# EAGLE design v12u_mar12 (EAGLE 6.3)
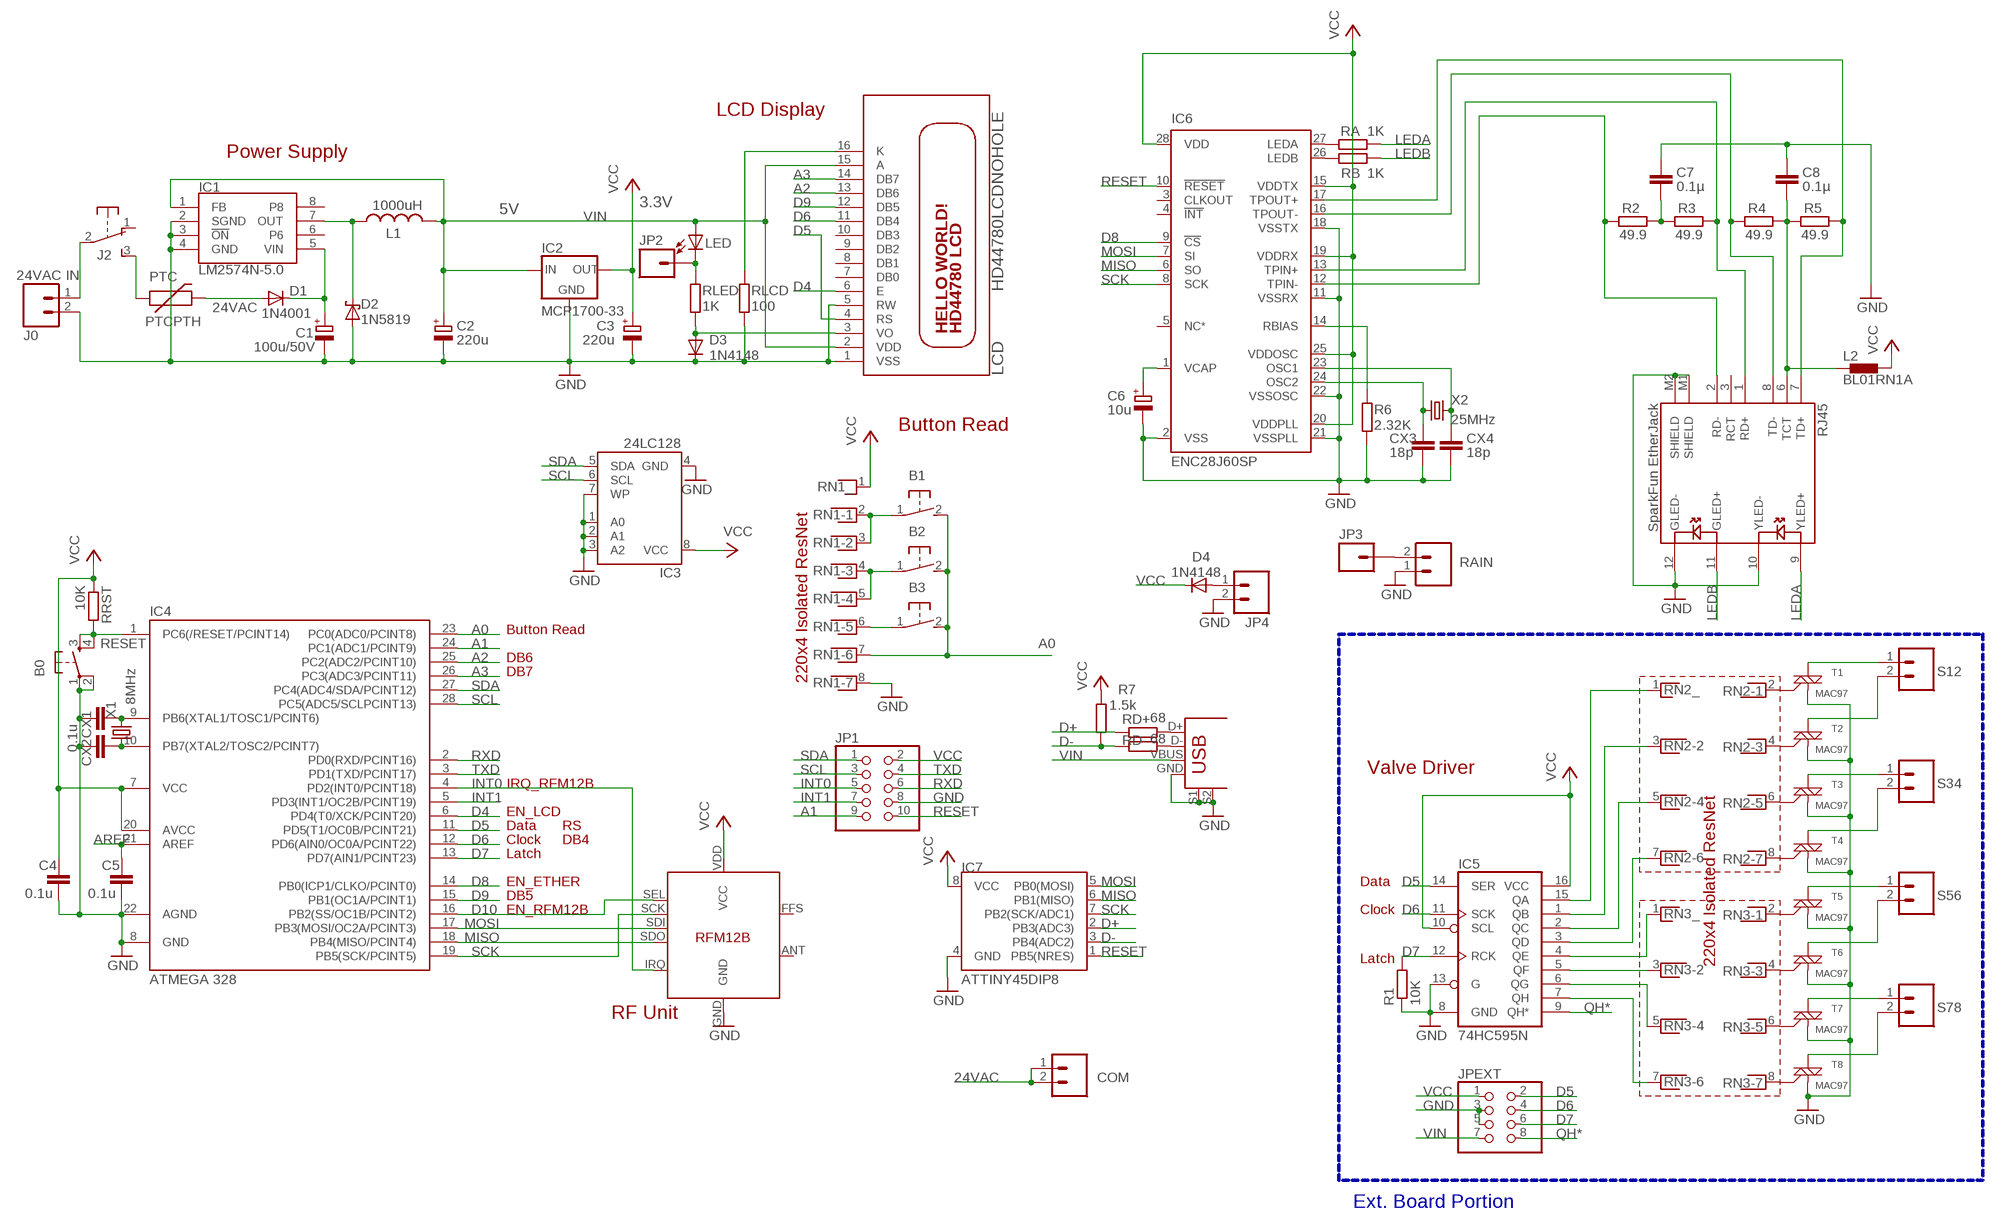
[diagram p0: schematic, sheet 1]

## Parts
B0  TAC_SWITCHPTH  [TACTILE-PTH]
B1  31-XX  [B3F-31XX]
B2  31-XX  [B3F-31XX]
B3  31-XX  [B3F-31XX]
C1  100u/50V  CPOL-EUE3.5-8  [E3,5-8]
C2  220u  CPOL-EUE2-5  [E2-5]
C3  220u  CPOL-EUE2-5  [E2-5]
C4  0.1u  C-EU025-024X044  [C025-024X044]
C5  0.1u  C-EU025-024X044  [C025-024X044]
C6  10u  CPOL-EUE1.8-4  [E1,8-4]
C7  0.1µ  C-EU025-024X044  [C025-024X044]
C8  0.1µ  C-EU025-024X044  [C025-024X044]
COM  M025MM  [SCREWTERMINAL-5MM-2]
CX1  0.1u  C-EU025-024X044  [C025-024X044]
CX2  0.1u  C-EU025-024X044  [C025-024X044]
CX3  18p  C-EU025-024X044  [C025-024X044]
CX4  18p  C-EU025-024X044  [C025-024X044]
D1  1N4001  DIODE-DO41-7.6  [DO41-7.6]
D2  1N5819  1N5817-B  [DO41-7.6]
D3  1N4148  1N4148DO35-7  [DO35-7]
D4  1N4148  1N4148DO35-7  [DO35-7]
IC1  LM2574N-5.0  LM2574N  [DIL08]
IC2  MCP1700-33  MCP1700INLINE  [TO92-INLINE]
IC3  24LC128  AT24CP  [DIL08]
IC4  ATMEGA 328  ATMEGA48/88/168-PU  [DIL28-3]
IC5  74HC595N  74LS595N  [DIL16]
IC6  ENC28J60SP  [DIL28-3]
IC7  ATTINY45DIP8  [DIP08]
IC8  RFM12B  [RFM12B]
J0  24VAC IN  M025MM  [SCREWTERMINAL-5MM-2]
J2  EG1206  [EG1206]
JP1  PINHD-2X5  [2X05]
JP2  M01PTH  [1X01]
JP3  M01PTH  [1X01]
JP4  M02PTH  [1X02]
JPEXT  PINHD-2X4  [2X04]
L1  1000uH  L-US6000-XXX-RC  [6000-XXXX-RC]
L2  BL01RN1A  [BL01RN1A]
LCD  HD44780LCDNOHOLE  [LCD1602A]
LED  POWERLED  LED3MM  [LED3MM]
PTC  PTCPTH  [PTC]
R1  10K  R-EU_0204/7  [0204/7]
R2  49.9  R-EU_0204/7  [0204/7]
R3  49.9  R-EU_0204/7  [0204/7]
R4  49.9  R-EU_0204/7  [0204/7]
R5  49.9  R-EU_0204/7  [0204/7]
R6  2.32K  R-EU_0204/7  [0204/7]
R7  1.5k  R-EU_0204/7  [0204/7]
RA  1K  R-EU_0204/7  [0204/7]
RAIN  M025MM  [SCREWTERMINAL-5MM-2]
RB  1K  R-EU_0204/7  [0204/7]
RD+  68  R-EU_0204/7  [0204/7]
RD-  68  R-EU_0204/7  [0204/7]
RJ45  SparkFun EtherJack  MAGJACK  [MAGJACK]
RLCD  100  R-EU_0204/7  [0204/7]
RLED  1K  R-EU_0204/7  [0204/7]
RN1  RNX7  [RN-8]
RN2  RNX7  [RN-8]
RN3  RNX7  [RN-8]
RRST  10K  R-EU_0204/7  [0204/7]
S12  M025MM  [SCREWTERMINAL-5MM-2]
S34  M025MM  [SCREWTERMINAL-5MM-2]
S56  M025MM  [SCREWTERMINAL-5MM-2]
S78  M025MM  [SCREWTERMINAL-5MM-2]
T1  MAC97  LX807DE  [TO-92]
T2  MAC97  LX807DE  [TO-92]
T3  MAC97  LX807DE  [TO-92]
T4  MAC97  LX807DE  [TO-92]
T5  MAC97  LX807DE  [TO-92]
T6  MAC97  LX807DE  [TO-92]
T7  MAC97  LX807DE  [TO-92]
T8  MAC97  LX807DE  [TO-92]
USB  USB+SHIELD  [USB-B-PTH]
X1  8MHz  CRYSTALTC26V  [TC26V]
X2  25MHz  CRYSTALHC49US  [HC49US]

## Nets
24VAC [power]: COM.1 COM.2 D1.A PTC.P$2
A0: B1.2(S) B2.2(S) B3.2(S) IC4.23(PC0(ADC0/PCINT8)) RN1.7
A1: IC4.24(PC1(ADC1/PCINT9)) JP1.9
A2: IC4.25(PC2(ADC2/PCINT10)) LCD.13(DB6)
A3: IC4.26(PC3(ADC3/PCINT11)) LCD.14(DB7)
AREF: C5.1 IC4.21(AREF)
D4: IC4.6(PD4(T0/XCK/PCINT20)) LCD.6(E)
D5: IC4.11(PD5(T1/OC0B/PCINT21)) IC5.14(SER) JPEXT.2 LCD.4(RS)
D6: IC4.12(PD6(AIN0/OC0A/PCINT22)) IC5.11(SCK) JPEXT.4 LCD.11(DB4)
D7: IC4.13(PD7(AIN1/PCINT23)) IC5.12(RCK) JPEXT.6 R1.2
D8: IC4.14(PB0(ICP1/CLKO/PCINT0)) IC6.9(!CS)
D9: IC4.15(PB1(OC1A/PCINT1)) LCD.12(DB5)
D10: IC4.16(PB2(SS/OC1B/PCINT2)) IC8.SEL
D+: IC7.2(PB3(ADC3)) RD+.1
D-: IC7.3(PB4(ADC2)) R7.1 RD-.1
GND [power]: B0.1 B0.2 C1.- C2.- C3.- C4.2 C5.2 C6.- C7.1 C8.1 CX1.1 CX2.1 CX3.2 CX4.2 D2.A D3.C IC1.2(SGND) IC1.3(!ON) IC1.4(GND) IC2.1(GND) IC3.1(A0) IC3.2(A1) IC3.3(A2) IC3.4(GND) IC3.7(WP) IC4.8(GND) IC4.22(AGND) IC5.8(GND) IC5.13(G) IC6.2(VSS) IC6.11(VSSRX) IC6.18(VSSTX) IC6.21(VSSPLL) IC6.22(VSSOSC) IC7.4(GND) IC8.GND J0.2 JP1.8 JP4.2 JPEXT.3 JPEXT.5 LCD.1(VSS) LCD.5(RW) R1.1 R6.2 RAIN.1 RJ45.10(YLED-) RJ45.12(GLED-) RJ45.M1(SHIELD) RJ45.M2(SHIELD) RLCD.2 RN1.8 T1.1(M1) T2.1(M1) T3.1(M1) T4.1(M1) T5.1(M1) T6.1(M1) T7.1(M1) T8.1(M1) USB.GND USB.S1 USB.S2
INT0: IC4.4(PD2(INT0/PCINT18)) IC8.IRQ JP1.5
INT1: IC4.5(PD3(INT1/OC2B/PCINT19)) JP1.7
LEDA: RA.2 RJ45.9(YLED+)
LEDB: RB.2 RJ45.11(GLED+)
MISO: IC4.18(PB4(MISO/PCINT4)) IC6.6(SO) IC7.6(PB1(MISO)) IC8.SDO
MOSI: IC4.17(PB3(MOSI/OC2A/PCINT3)) IC6.7(SI) IC7.5(PB0(MOSI)) IC8.SDI
N$2: CX1.2 IC4.9(PB6(XTAL1/TOSC1/PCINT6)) X1.2
N$3: RN2.2 T1.2(G)
N$4: IC5.5(QF) RN3.3
N$5: IC5.6(QG) RN3.5
N$6: J0.1 J2.2(P)
N$7: IC5.7(QH) RN3.7
N$8: CX2.2 IC4.10(PB7(XTAL2/TOSC2/PCINT7)) X1.1
N$9: C1.+ D1.C IC1.5(VIN)
N$10: IC5.4(QE) RN3.1
N$11: IC5.3(QD) RN2.7
N$12: IC5.2(QC) RN2.5
N$13: IC5.1(QB) RN2.3
N$14: IC5.15(QA) RN2.1
N$15: RN2.4 T2.2(G)
N$16 [power]: S12.1 T1.3(M2)
N$17 [power]: S12.2 T2.3(M2)
N$18 [power]: S34.1 T3.3(M2)
N$19: RN2.6 T3.2(G)
N$20 [power]: S34.2 T4.3(M2)
N$21: RN2.8 T4.2(G)
N$22 [power]: S56.1 T5.3(M2)
N$23 [power]: S56.2 T6.3(M2)
N$24 [power]: S78.1 T7.3(M2)
N$25 [power]: S78.2 T8.3(M2)
N$26: RN3.2 T5.2(G)
N$27: RN3.4 T6.2(G)
N$28: RN3.6 T7.2(G)
N$29: RN3.8 T8.2(G)
N$30: C8.2 L2.1 R4.2 R5.1 RJ45.6(TCT)
N$31: J2.3(S) PTC.P$1
N$32: B1.1(P) RN1.2 RN1.3
N$33: B3.1(P) RN1.6
N$34: IC6.27(LEDA) RA.1
N$35: B2.1(P) RN1.4 RN1.5
N$36: IC6.26(LEDB) RB.1
N$37: JP2.1 LED.K(C) RLED.1
N$38: RD+.2 USB.D+
N$39: D3.A LCD.3(VO) RLED.2
N$40 [power]: D2.C IC1.7(OUT) L1.1
N$41: IC6.17(TPOUT+) R5.2 RJ45.7(TD+)
N$42: IC6.16(TPOUT-) R4.1 RJ45.8(TD-)
N$43: IC6.13(TPIN+) R3.2 RJ45.1(RD+)
N$44: IC6.12(TPIN-) R2.1 RJ45.2(RD-)
N$45: RD-.2 USB.D-
N$46: D4.A JP4.1
N$47: JP3.1 RAIN.2
N$48: LCD.16(K) RLCD.1
N$50: C6.+ IC6.1(VCAP)
N$51: IC6.14(RBIAS) R6.1
N$52: CX3.1 IC6.24(OSC2) X2.1
N$53: CX4.1 IC6.23(OSC1) X2.2
N$54: C7.2 R2.2 R3.1
QH*: IC5.9(QH*) JPEXT.8
RESET: B0.3 B0.4 IC4.1(PC6(/RESET/PCINT14)) IC6.10(!RESET) IC7.1(PB5(NRES)) JP1.10 RRST.2
RXD: IC4.2(PD0(RXD/PCINT16)) JP1.6
SCK: IC4.19(PB5(SCK/PCINT5)) IC6.8(SCK) IC7.7(PB2(SCK/ADC1)) IC8.SCK
SCL: IC3.6(SCL) IC4.28(PC5(ADC5/SCLPCINT13)) JP1.3
SDA: IC3.5(SDA) IC4.27(PC4(ADC4/SDA/PCINT12)) JP1.1
TXD: IC4.3(PD1(TXD/PCINT17)) JP1.4
VCC: C3.+ C4.1 D4.C IC2.3(OUT) IC3.8(VCC) IC4.7(VCC) IC4.20(AVCC) IC5.10(SCL) IC5.16(VCC) IC6.15(VDDTX) IC6.19(VDDRX) IC6.20(VDDPLL) IC6.25(VDDOSC) IC6.28(VDD) IC7.8(VCC) IC8.VDD(VCC) JP1.2 JPEXT.1 L2.2 R7.2 RN1.1 RRST.1
VIN: C2.+ IC1.1(FB) IC2.2(IN) JPEXT.7 L1.2 LCD.2(VDD) LCD.15(A) LED.A USB.VBUS
Unconnected: IC1.6 IC1.8 IC6.3(CLKOUT) IC6.4(!INT) IC6.5(NC*) IC8.ANT IC8.FFS J2.1(O) LCD.7(DB0) LCD.8(DB1) LCD.9(DB2) LCD.10(DB3) RJ45.3(RCT)

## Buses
B$1

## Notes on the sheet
- LCD Display
- Power Supply
- 3.3V
- 5V
- Button Read
- Button Read
- DB6
- DB7
- 220x4 Isolated ResNet
- Valve Driver
- IRQ_RFM12B
- 220x4 Isolated ResNet
- EN_LCD
- Data | RS
- Clock | DB4
- Latch
- EN_ETHER | Data
- DB5
- EN_RFM12B | Clock
- Latch
- RF Unit
- Ext. Board Portion

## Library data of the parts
B0 = SparkFun:TAC_SWITCH: Momentary Switch Button commonly used for reset or general input. Spark Fun Electronics SKU : COM-00097
B1-B3 = adafruit:31-XX: OMRON SWITCH
C1-C3 C6 = resistor:CPOL-EU: POLARIZED CAPACITOR, European symbol
C4 C5 CX1 CX2 = rcl:C-EU: CAPACITOR, European symbol
C7 C8 CX3 CX4 = resistor:C-EU: CAPACITOR, European symbol
COM J0 JP4 RAIN S12 S34 S56 S78 = SparkFun:M02: Header 2
D1 = diode:DIODE-: DIODE
D2 = diode:1N581*: 1.0A SCHOTTKY BARRIER RECTIFIER
D3 D4 = diode:1N4148: DIODE
IC1 = linear-technology:LM2574N
IC2 = adafruit:MCP1700: VOLTAGE REGULATOR
IC3 = atmel:AT24C*: 2-wire serial EEPROM; MPN: AT24C1024BW-SH-B; OC_FARNELL: 1362646; OC_NEWARK: 03P2044
IC4 = atmega8:ATMEGA48/88/168-PU
IC5 = SparkFun:74*595: 8-bit SHIFT REGISTER, output latch
IC6 = microchip:ENC28J60: Stand-Alone Ethernet Controller with SPI Interface Source: http://ww1.microchip.com/downloads/en/DeviceDoc/39662c.pdf; MF: MICROCHIP; MPN: ENC28J60/SP; OC_FARNELL: 1084619; OC_NEWARK: 96K3661
IC7 = SparkFun:ATTINY45: Atmel ATTiny45
IC8 = JeeLabs:RFM12B
J2 = adafruit:EG1206
JP1 = pinhead:PINHD-2X5: PIN HEADER
JP2 JP3 = SparkFun:M01: Header 1
JPEXT = pinhead:PINHD-2X4: PIN HEADER
L1 = rcl:L-US: INDUCTOR, American symbol
L2 = inductors:BL0: Noise Suppression Products/EMI Suppression Filters, Lead EMIFIL(R) Inductor Type
LCD = adafruit:HD44780LCD: HD44780 LCD Standard character type LCDs, available in sizes from 8x1 to 40x4!
LED = adafruit:LED: LED
PTC = SparkFunNew:PTC: Resettable Fuse PTC
R1-R7 RA RB RD+ RD- RLCD RLED RRST = rcl:R-EU_: RESISTOR, European symbol
RJ45 = SparkFunNew:MAGJACK
RN1-RN3 = resistor-net:RNX7: RESISTOR NETWORK; OC_FARNELL: unknown; OC_NEWARK: unknown
T1-T8 = SparkFun:LX807DE: LX807DE Triac http://www.littelfuse.com/data/en/Data_Sheets/Littelfuse_Triac_LX8.pdf
USB = SparkFunNew:USB+SHIELD: USB+Shield USB connector with shield pins connectable
X1 = crystal:CRYSTAL: CRYSTAL; OC_FARNELL: unknown; OC_NEWARK: unknown
X2 = SparkFun:CRYSTAL: Crystals

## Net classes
0 default: width 0.406 mm, clearance 0.203 mm
1 power: width 0.813 mm, clearance 0.203 mm

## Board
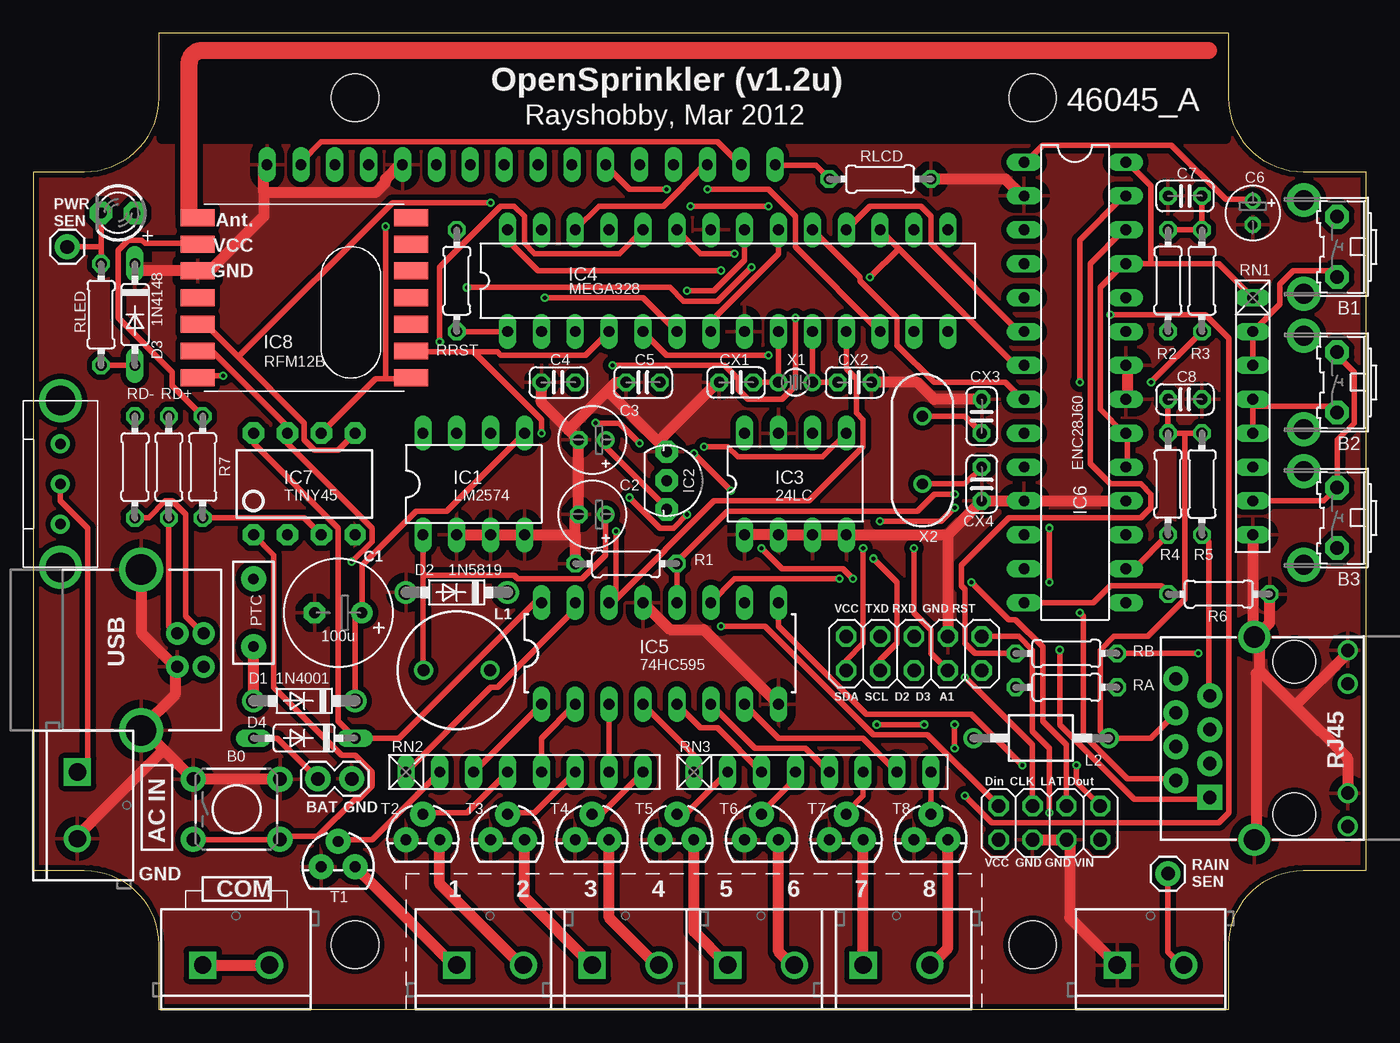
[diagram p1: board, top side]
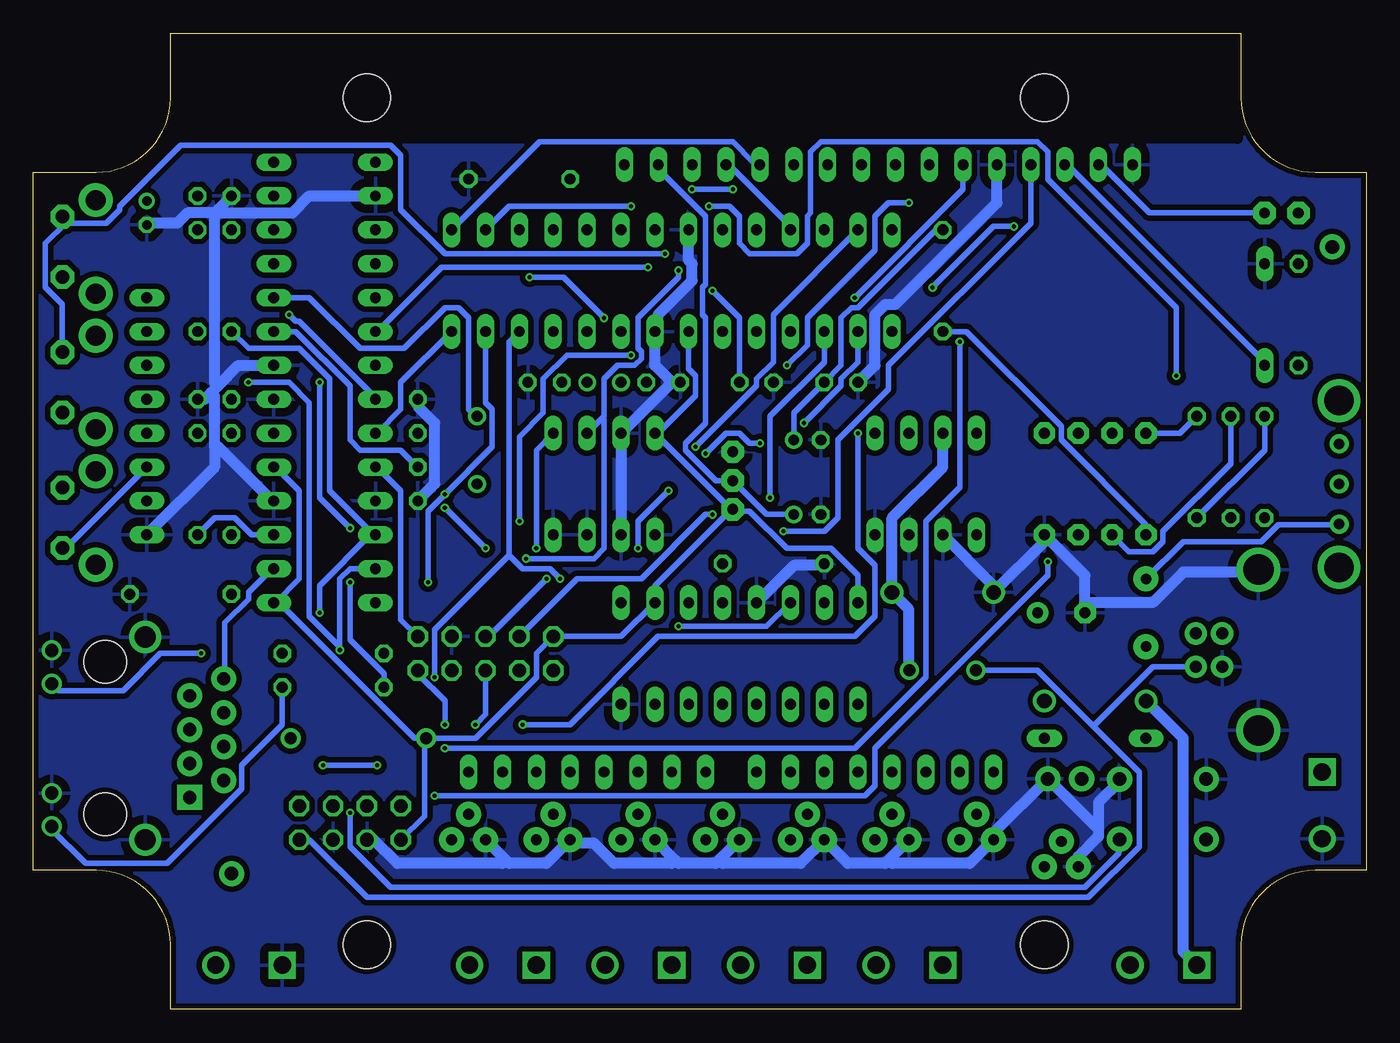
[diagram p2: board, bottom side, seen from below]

Size 99.95 x 73.15 mm. Coordinates in mm from the lower left corner, seen from the top.
Outline: 9.4,0 89.66,0 89.66,4.83 arc-90 95.25,10.41 99.95,10.41 99.95,62.74 95.25,62.74 arc-90 89.66,68.33 89.66,73.15 9.4,73.15 9.4,68.33 arc-90 3.81,62.74 0,62.74 0,10.41 3.81,10.41 arc-90 9.4,4.83 9.4,0
Copper layers (1*16): Top 0.035mm / dielectric 1.5mm / Bottom 0.035mm
Design rules "Fusion_eagle_rule_v1.1 *": minimum track width 6mil, minimum drill 12mil, track to track 6mil, track to pad 6mil, pad to pad 8mil, via to via 8mil, smd to smd 0mil, copper to edge 10mil, drill to drill 10mil, minimum pad ring 10mil, minimum via ring 6mil, stop-mask expansion 2mil, vias tented up to drill 100mil, thermal gap 25mil
Holes 3.56 mm at 24.13,4.83 74.93,4.83 24.13,68.33 74.93,68.33
tRestrict: area 9.7,65.3 to 89.4,72.6
bRestrict: area 9.7,65.3 to 89.4,72.6
vRestrict: area 21.6,2.3 to 26.7,7.4; area 72.4,2.3 to 77.5,7.4; area 71.1,16.8 to 81.3,17.5; area 71.1,10.7 to 81.3,11.4; area 64.8,36.8 to 68.6,47; area 59.9,29.5 to 71.9,30.5; area 59.9,22.9 to 71.9,23.9; area 86.9,9.1 to 89.7,11.2; area 8.4,12.2 to 10.2,18; area 7.9,9.7 to 10.4,10.7; area 1.5,58.7 to 3.6,60.7

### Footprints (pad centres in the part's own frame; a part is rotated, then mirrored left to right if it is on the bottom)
TACTILE-PTH = drill 1.016 pad 1.88: 1 -3.251,2.261; 2 3.251,2.261; 3 -3.251,-2.261; 4 3.251,-2.261
B3F-31XX = drill 1.016 pad 1.778 octagon: 1 -2.261,-1.245; 2 2.261,-1.245 | drill 1.499 pad 2.54: 3 -3.505,1.245; 4 3.505,1.245
E3,5-8 = drill 0.813 pad 1.6: + -1.778,0 | drill 0.813 pad 1.6 octagon: - 1.778,0
E2-5 = drill 0.813 pad 1.27: + -1.016,0 | drill 0.813 pad 1.27 octagon: - 1.016,0
C025-024X044 = drill 0.813 octagon: 1 -1.27,0; 2 1.27,0
E1,8-4 = drill 0.711 pad 1.168: + -0.889,0 | drill 0.711 pad 1.168 octagon: - 0.889,0
SCREWTERMINAL-5MM-2 = drill 1.3 pad 2.032 square: 1 0,0 | drill 1.3 pad 2.032: 2 5,0
DO41-7.6 = drill 1.1 pad 1.7: A 3.81,0; C -3.81,0
DO35-7 = drill 0.813 long: A 3.81,0; C -3.81,0
DIL08 = drill 0.813 long: 1 -3.81,-3.81; 2 -1.27,-3.81; 3 1.27,-3.81; 4 3.81,-3.81; 5 3.81,3.81; 6 1.27,3.81; 7 -1.27,3.81; 8 -3.81,3.81
TO92-INLINE = drill 0.813 pad 1.676 octagon: 1 -2.159,0; 2 0,0; 3 2.159,0
DIL28-3 = drill 0.813 long: 1 -16.51,-3.81; 2 -13.97,-3.81; 3 -11.43,-3.81; 4 -8.89,-3.81; 5 -6.35,-3.81; 6 -3.81,-3.81; 7 -1.27,-3.81; 8 1.27,-3.81; 9 3.81,-3.81; 10 6.35,-3.81; 11 8.89,-3.81; 12 11.43,-3.81; 13 13.97,-3.81; 14 16.51,-3.81; 15 16.51,3.81; 16 13.97,3.81; 17 11.43,3.81; 18 8.89,3.81; 19 6.35,3.81; 20 3.81,3.81; 21 1.27,3.81; 22 -1.27,3.81; 23 -3.81,3.81; 24 -6.35,3.81; 25 -8.89,3.81; 26 -11.43,3.81; 27 -13.97,3.81; 28 -16.51,3.81
DIL16 = drill 0.813 long: 1 -8.89,-3.81; 2 -6.35,-3.81; 3 -3.81,-3.81; 4 -1.27,-3.81; 5 1.27,-3.81; 6 3.81,-3.81; 7 6.35,-3.81; 8 8.89,-3.81; 9 8.89,3.81; 10 6.35,3.81; 11 3.81,3.81; 12 1.27,3.81; 13 -1.27,3.81; 14 -3.81,3.81; 15 -6.35,3.81; 16 -8.89,3.81
DIP08 = drill 0.813 pad 1.6 octagon: 1 -3.81,-3.81; 2 -1.27,-3.81; 3 1.27,-3.81; 4 3.81,-3.81; 5 3.81,3.81; 6 1.27,3.81; 7 -1.27,3.81; 8 -3.81,3.81
RFM12B = smd 2.54 x 1.27: ANT 8,-6; FFS -8,2; GND 8,-2; IRQ -8,4; P$8 -8,0; P$9 -8,-2; P$10 -8,-4; P$12 -8,-6; P$16 8,0; SCK 8,4; SDI 8,2; SDO -8,6; SEL 8,6; VDD 8,-4
EG1206 = drill 0.8 pad 1.422: 1 -3,0; 2 0,0; 3 3,0 | drill 2.2: MT1 -6.25,0; MT2 6.25,0
2X05 = drill 1.016 octagon: 1 -5.08,-1.27; 2 -5.08,1.27; 3 -2.54,-1.27; 4 -2.54,1.27; 5 0,-1.27; 6 0,1.27; 7 2.54,-1.27; 8 2.54,1.27; 9 5.08,-1.27; 10 5.08,1.27
1X01 = drill 1.016 pad 1.88: 1 0,0
1X02 = drill 1.016 pad 1.88: 1 0,0; 2 2.54,0
2X04 = drill 1.016 octagon: 1 -3.81,-1.27; 2 -3.81,1.27; 3 -1.27,-1.27; 4 -1.27,1.27; 5 1.27,-1.27; 6 1.27,1.27; 7 3.81,-1.27; 8 3.81,1.27
6000-XXXX-RC = drill 0.9 pad 1.422: 1 -2.5,0; 2 2.5,0
BL01RN1A = drill 0.9 pad 1.5: 1 -5.08,0; 2 5.08,0
LCD1602A = drill 0.8 long: 1 8,33.46; 2 10.54,33.46; 3 13.08,33.46; 4 15.62,33.46; 5 18.16,33.46; 6 20.7,33.46; 7 23.24,33.46; 8 25.78,33.46; 9 28.32,33.46; 10 30.86,33.46; 11 33.4,33.46; 12 35.94,33.46; 13 38.48,33.46; 14 41.02,33.46; 15 43.56,33.46; 16 46.1,33.46
LED3MM = drill 0.813 pad 1.676 octagon: A -1.27,0; K 1.27,0
PTC = drill 0.8 pad 1.88: P$1 -2.54,0; P$2 2.54,0
0204/7 = drill 0.813 octagon: 1 -3.81,0; 2 3.81,0
MAGJACK = drill 1 pad 1.88 square: 1 3.175,17.445 | drill 1 pad 1.88: 2 4.445,19.985; 3 5.715,17.445; 4 6.985,19.985; 5 8.255,17.445; 6 9.525,19.985; 7 10.795,17.445; 8 12.065,19.985 | drill 1 pad 1.27: 9 1,7.1; 10 3.5,7.1; 11 11.7,7.1; 12 14.2,7.1 | drill 1.6 pad 2.184: M1 0,14.1; M2 15.2,14.1 | hole 3.2: 1.905,11.095; 13.335,11.095
RN-8 = drill 0.813 long: 1 -8.89,0; 2 -6.35,0; 3 -3.81,0; 4 -1.27,0; 5 1.27,0; 6 3.81,0; 7 6.35,0; 8 8.89,0
TO-92 = drill 0.813 pad 1.88: 1 -1.27,0; 2 0,1.905; 3 1.27,0
USB-B-PTH = drill 0.914 pad 1.676: D+ 0,1.25; D- 1.981,1.25; GND 0,-1.25; VBUS 1.981,-1.25 | drill 2.286: S1 -2.718,-6.02; S2 -2.718,6.02
TC26V = drill 0.813: 1 -1.27,0; 2 1.27,0
HC49US = drill 0.813: 1 -2.54,0; 2 2.54,0

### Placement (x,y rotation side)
B0  15.24,14.99 0 top
B1  96.52,57.15 90 top
B2  96.52,46.99 90 top
B3  96.52,36.83 90 top
C1  22.86,29.72 180 top
C2  41.91,37.08 180 top
C3  41.91,42.67 180 top
C4  39.37,46.99 180 top
C5  45.72,46.99 180 top
C6  91.44,59.69 270 top
C7  86.36,60.96 0 top
C8  86.36,45.72 180 top
COM  12.7,3.3 0 top
CX1  52.7,46.99 0 top
CX2  61.59,46.99 180 top
CX3  71.12,44.45 90 top
CX4  71.12,39.37 270 top
D1  20.32,23.11 180 top
D2  31.75,31.24 180 top
D3  7.62,52.07 270 top
D4  20.32,20.32 180 top
IC1  33.02,39.37 0 top
IC2  47.5,39.62 270 top
IC3  57.15,39.37 0 top
IC4  52.07,54.61 0 top
IC5  46.99,26.67 0 top
IC6  78.11,46.99 270 top
IC7  20.32,39.37 0 top
IC8  20.32,53.34 180 top
J0  3.3,17.78 270 top
J2  2.03,39.37 270 top
JP1  66.04,26.67 0 top
JP2  2.54,57.15 0 top
JP3  85.09,10.16 0 top
JP4  21.34,17.27 0 top
JPEXT  76.2,13.97 0 top
L1  31.75,25.4 180 top
L2  75.56,20.32 180 top
LCD  9.53,29.84 0 top
LED  6.35,59.69 180 top
PTC  16.51,29.72 270 top
R1  44.45,33.4 0 top
R2  85.09,54.61 90 top
R3  87.63,54.61 270 top
R4  85.09,39.37 90 top
R5  87.63,39.37 270 top
R6  88.9,31.11 0 top
R7  12.7,40.64 90 top
RA  77.47,24.13 0 top
RAIN  81.28,3.3 0 top
RB  77.47,26.67 0 top
RD+  10.16,40.64 270 top
RD-  7.62,40.64 270 top
RJ45  105.66,12.7 90 top
RLCD  63.5,62.23 0 top
RLED  5.08,52.07 270 top
RN1  91.44,44.45 270 top
RN2  36.83,17.78 0 top
RN3  58.42,17.78 0 top
RRST  31.75,54.61 270 top
S12  31.75,3.3 0 top
S34  41.91,3.3 0 top
S56  52.07,3.3 0 top
S78  62.23,3.3 0 top
T1  22.86,10.67 0 top
T2  29.21,12.7 0 top
T3  35.56,12.7 0 top
T4  41.91,12.7 0 top
T5  48.26,12.7 0 top
T6  54.61,12.7 0 top
T7  60.96,12.7 0 top
T8  67.31,12.7 0 top
USB  10.79,26.92 0 top
X1  57.15,46.99 180 top
X2  66.67,41.91 270 top

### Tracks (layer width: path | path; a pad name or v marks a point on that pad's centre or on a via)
24VAC
  Top 0.813: D1.A PTC.P$2 | COM.1 COM.2
  Bottom 0.813: D1.A 13.72,20.32 13.72,4.32 COM.1
A0  (via drill 0.3)
  Top 0.406: RN1.7 96.77,38.1 B3.2 97.79,39.12 97.79,42.67 99.06,43.94 99.06,47.75 97.79,49.02 B2.2 | IC4.23 50.04,56.64 v52.58,56.64
  Bottom 0.406: v52.58,56.64 69.09,56.64 72.39,59.94 72.39,64.01 73.15,64.77 88.9,64.77 93.47,60.2 93.47,59.94 94.49,58.93 97.28,58.93 B1.2 97.54,58.93 99.06,57.4 99.06,54.1 97.79,52.83 97.79,49.28 B2.2
A1  (via drill 0.3)
  Top 0.406: IC4.24 43.94,56.64 37.59,56.64 36.83,57.4 36.83,59.44 36.07,60.2 35.05,60.2 30.48,55.63 v30.48,50.04 | v69.09,19.56 v69.09,21.34
  Bottom 0.406: v30.48,50.04 30.48,39.12 33.02,36.58 33.02,24.89 38.35,19.56 v69.09,19.56 | v69.09,21.34 69.09,23.11 71.12,25.15 JP1.9
A2
  Bottom 0.406: IC4.25 43.18,58.67 47.75,63.25 LCD.13
A3
  Top 0.406: IC4.26 42.42,60.2 47.24,60.2 50.29,63.25 LCD.14
AREF  (via drill 0.3)
  Top 0.406: v49.02,53.85 51.05,53.85 53.34,56.13 IC4.21
  Bottom 0.406: C5.1 46.99,51.82 v49.02,53.85
D4  (via drill 0.3)
  Top 0.406: v38.35,53.34 45.72,53.34 IC4.6
  Bottom 0.406: v38.35,53.34 30.23,61.47 30.23,63.25 LCD.6
D5  (via drill 0.3)
  Top 0.406: v43.69,35.81 43.69,30.99 IC5.14 43.69,30.73 51.05,38.1 58.17,38.1 62.23,42.16 62.23,44.2 61.72,44.7 61.72,47.24 60.96,48.01 IC4.11 | JPEXT.2 67.06,20.57 62.99,20.57 54.86,28.7 v51.56,28.7
  Bottom 0.406: v43.69,35.81 40.64,35.81 39.62,36.83 39.62,42.67 35.81,46.48 35.81,48.26 25.15,58.93 25.15,63.25 LCD.4 | v51.56,28.7 44.96,28.7 IC5.14
D6  (via drill 0.3)
  Top 0.406: v47.5,61.47 44.7,61.47 42.93,63.25 LCD.11 | v50.55,61.47 55.12,61.47 57.15,59.44 57.15,57.15 IC4.12 | IC5.11 52.58,32.26 v60.45,32.26 | JPEXT.4 74.93,19.81 v69.85,24.89
  Bottom 0.406: v50.55,61.47 v47.5,61.47 | v60.45,32.26 61.21,33.02 63.25,33.02 64.26,34.04 | 64.26,34.04 64.26,50.04 IC4.12 | v69.85,24.89 69.85,28.45 64.26,34.04
D7  (via drill 0.3)
  Top 0.406: IC5.12 R1.2 48.26,33.53 52.07,37.34 66.29,37.34 67.56,38.61 v69.09,38.61 | JPEXT.6 77.47,19.81 75.69,21.59 75.69,27.18 73.66,29.21 73.15,29.21 v70.36,32
  Bottom 0.406: IC4.13 66.04,45.47 65.53,44.96 65.53,42.16 v69.09,38.61 70.36,37.34 v70.36,32
D8
  Bottom 0.406: IC4.14 72.39,46.99 72.39,44.96 74.17,43.18 IC6.9
D9
  Bottom 0.406: IC4.15 61.98,65.02 47.5,65.02 45.97,63.5 45.47,63.5 LCD.12
D10  (via drill 0.3)
  Top 0.406: v14.22,47.5 12.45,47.5 IC8.SEL | v49.28,60.2 v55.12,60.2
  Bottom 0.406: v14.22,47.5 14.22,52.58 23.88,62.23 23.88,64.26 24.64,65.02 40.89,65.02 41.66,64.26 41.66,59.69 41.91,59.44 41.91,57.4 42.67,56.64 46.23,56.64 46.99,57.4 46.99,59.44 47.75,60.2 v49.28,60.2 | v55.12,60.2 64.26,60.2 IC4.16
D+
  Bottom 0.406: RD+.1 10.16,40.89 15.24,35.81 15.24,35.05 16,34.29 17.78,34.29 IC7.2
D-
  Top 0.406: R7.1 20.32,36.83 IC7.3
  Bottom 0.406: RD-.1 7.62,41.91 R7.1
GND
  Top 0.813: 9.78,19.43 8.38,20.83 USB.S1 8.13,21.08 10.67,23.62 10.67,25.65 USB.GND 10.41,25.91 8.13,28.19 8.13,32.77 USB.S2 | 9.78,19.43 11.94,17.27 B0.1 12.19,17.27 18.29,17.27 B0.2 | J0.2 3.3,12.95 9.78,19.43 | JPEXT.3 JPEXT.5 77.72,12.45 77.72,6.86 RAIN.1 | D3.C 8.13,55.37 12.19,55.37 IC8.GND 12.7,55.37 13.21,55.37 17.27,59.44 17.27,61.21 | 17.27,61.21 17.27,63.25 LCD.1 | LCD.5 27.43,63.25 26.42,62.23 26.42,61.98 25.65,61.21 17.27,61.21 | IC1.2 IC1.3 IC1.4 40.64,35.56 | 40.64,35.56 40.64,36.83 C2.- C3.- 40.13,43.43 | 40.64,35.56 R1.1 | IC5.8 50.29,28.45 47.75,28.45 IC5.13 | C4.2 38.1,45.47 40.13,43.43 | C5.2 43.69,46.99 43.05,46.35 | 40.13,43.43 43.05,46.35 | 46.86,42.55 47.5,41.91 IC2.1 | 43.05,46.35 46.86,42.55 | CX1.1 51.31,46.99 46.86,42.55 | CX3.2 67.56,45.72 66.29,46.99 CX2.1 | IC3.1 IC3.2 IC3.3 IC3.4 68.58,35.56 | IC6.18 IC6.11 CX4.2 68.58,35.56 | 68.58,35.56 JP1.8 | R6.2 92.71,28.96 91.69,27.94 RJ45.M2 | RN1.8 91.44,28.19 RJ45.M2 | 91.95,25.4 94.61,22.73 | 94.61,22.73 98.55,18.8 98.55,16.26 RJ45.10 | 91.95,25.4 91.95,27.69 RJ45.M2 | RJ45.12 98.55,26.67 94.61,22.73 | RJ45.M1 91.69,12.7 91.69,25.15 91.95,25.4 | RLCD.2 72.9,62.23 74.17,60.96 IC6.2 | IC6.21 82.04,45.72 82.04,48.26 IC6.22
  Bottom 0.813: T1.1 21.59,11.43 20.07,12.95 20.07,13.72 | 20.07,13.72 20.07,15.49 18.54,17.02 B0.2 | 20.07,13.72 20.32,13.72 JP4.2 27.94,13.21 T2.1 29.72,10.92 35.56,10.92 35.81,11.18 | 64.52,11.18 T8.1 | 64.52,11.18 64.26,10.92 61.47,10.92 T7.1 59.44,12.45 57.91,12.45 56.39,10.92 52.07,10.92 51.82,11.18 | 35.81,11.18 36.07,10.92 38.86,10.92 T4.1 42.42,10.92 48.26,10.92 48.51,11.18 | 35.81,11.18 T3.1 | 48.51,11.18 48.77,10.92 51.56,10.92 51.82,11.18 | 48.51,11.18 T5.1 | 51.82,11.18 T6.1 | JPEXT.3 74.42,12.7 72.64,10.92 64.77,10.92 64.52,11.18 | 52.07,46.99 IC3.7 IC3.2 | CX1.1 52.07,46.99 | 52.07,46.99 53.34,48.26 IC4.8 53.09,51.05 53.09,52.07 50.55,54.61 50.55,55.88 50.8,56.13 IC4.22 | IC5.13 42.93,33.27 40.64,33.27 R1.1 | IC1.2 27.94,31.75 D2.A 24.13,35.05 IC7.4 21.08,32.51 C1.- 20.83,30.48 16,30.48 13.72,32.77 8.13,32.77 USB.S2 | C4.2 36.83,48.26 36.83,52.07 36.07,52.83 35.31,52.83 27.69,60.45 27.69,63.25 LCD.5 | CX3.2 71.12,45.21 69.85,43.94 69.85,39.37 CX4.2 | 86.36,59.69 88.39,59.69 89.15,58.93 91.44,58.93 C6.- | 86.11,59.94 C7.1 | 86.36,59.69 86.11,59.94 | C8.1 87.12,45.72 86.61,46.23 | 86.11,46.74 84.58,48.26 IC6.22 | 86.61,46.23 86.11,46.74 | 86.36,59.69 86.36,46.99 86.11,46.74 | IC6.2 79.25,60.96 80.52,59.69 85.85,59.69 86.11,59.94 | RN1.8 86.36,40.64 86.36,42.16 | 86.36,42.16 86.36,45.97 86.61,46.23 | IC6.18 82.04,38.1 86.11,42.16 86.36,42.16
  pour Top (isolate 0.406): 0,73.66 100.33,73.66 100.33,0 0,0
  pour Bottom (isolate 0.406): 0,73.66 100.33,73.66 100.33,0 0,0
INT0  (via drill 0.3)
  Top 0.406: 33.02,49.28 34.8,49.28 35.05,49.02 41.4,49.02 IC4.4 | 33.02,49.28 28.45,49.28 IC8.IRQ | v63.25,21.34 v66.8,21.34 | v38.1,43.18 38.1,44.2 33.02,49.28
  Bottom 0.406: JP1.5 66.04,22.1 v66.8,21.34 | v63.25,21.34 59.69,21.34 53.09,27.94 38.35,27.94 36.83,29.46 36.83,33.27 38.1,34.54 v38.1,43.18
INT1  (via drill 0.3)
  Top 0.406: IC4.5 47.5,49.02 v55.12,49.02 | v63.5,36.58 68.07,36.58 v69.09,37.59 | v66.04,34.54 66.04,29.72 67.31,28.45 67.31,26.67 JP1.7
  Bottom 0.406: v55.12,49.02 59.94,49.02 61.72,47.24 61.72,44.7 63.5,42.93 v63.5,36.58 | v66.04,34.54 v69.09,37.59
LEDA
  Bottom 0.406: RA.2 81.28,21.34 84.33,18.29 84.33,16.51 89.92,10.92 96.01,10.92 98.55,13.46 RJ45.9
LEDB  (via drill 0.3)
  Top 0.406: RB.2 v87.38,26.67
  Bottom 0.406: v87.38,26.67 90.42,26.67 93.22,23.88 98.04,23.88 98.55,24.38 RJ45.11
MISO  (via drill 0.3)
  Top 0.406: 26.42,47.24 25.65,47.24 IC7.6 | 26.42,47.24 28.19,47.24 IC8.SDO | IC4.18 62.74,60.2 66.55,60.2 67.31,59.44 67.31,57.4 73.91,50.8 IC6.6 | 26.42,47.24 v26.42,58.67 | v32.51,54.1 47.75,54.1 48.77,53.09 51.31,53.09 v53.85,55.63
  Bottom 0.406: v26.42,58.67 27.94,58.67 v32.51,54.1 | v53.85,55.63 69.34,55.63 74.17,50.8 IC6.6
MOSI  (via drill 0.3)
  Top 0.406: 15.37,48.9 20.32,43.94 20.32,42.67 21.08,41.91 22.86,41.91 IC7.5 | 15.37,48.9 12.95,51.31 12.45,51.31 IC8.SDI | 64.9,57.02 IC4.17 | 64.9,57.02 73.66,48.26 IC6.7 | v34.29,60.45 26.92,60.45 15.37,48.9 | v43.43,48.26 51.82,48.26 52.83,47.24 52.83,46.48 53.59,45.72 56.13,45.72 57.15,46.74 v57.15,51.82 | v62.74,54.86 64.9,57.02
  Bottom 0.406: v34.29,60.45 35.81,60.45 36.83,59.44 36.83,56.9 41.91,51.82 41.91,49.78 v43.43,48.26 | v57.15,51.82 60.2,54.86 v62.74,54.86
N$1
  Top 1.27: 11.68,59.69 11.68,70.87 arc-90 12.7,71.88 88.14,71.88
N$2
  Top 0.406: CX1.2 X1.2 IC4.9
N$3
  Top 0.406: RN2.2 25.4,12.7 22.86,12.7 T1.2
N$4
  Top 0.406: RN3.3 51.31,21.08 50.04,21.08 IC5.5
N$5
  Top 0.406: IC5.6 54.1,19.56 57.91,19.56 RN3.5
N$6
  Top 0.406: J2.2 2.03,38.1 4.06,36.07 4.06,18.54 J0.1
N$7
  Top 0.406: IC5.7 55.88,20.32 62.23,20.32 RN3.7
N$8
  Top 0.406: CX2.2 X1.1 IC4.10
N$9
  Top 0.406: IC1.5 30.99,37.34 28.7,37.34 24.64,33.27 C1.+ 24.13,29.21 D1.C
N$10
  Top 0.406: RN3.1 49.53,19.05 IC5.4
N$11
  Top 0.406: RN2.7 IC5.3
N$12
  Top 0.406: RN2.5 38.1,20.32 IC5.2
N$13
  Top 0.406: RN2.3 IC5.1
N$14
  Top 0.406: RN2.1 34.29,24.13 34.8,24.13 40.64,29.97 IC5.15
N$15
  Top 0.406: RN2.4 32.51,14.73 29.21,14.73 T2.2
N$16
  Top 0.813: T1.3 31.5,3.3 S12.1
N$17
  Top 0.813: T2.3 30.48,9.4 36.58,3.3 S12.2
N$18
  Top 0.813: T3.3 36.83,8.38 S34.1
N$19
  Top 0.406: RN2.6 37.59,14.73 35.56,14.73 T3.2
N$20
  Top 0.813: T4.3 43.18,6.86 46.74,3.3 S34.2
N$21
  Top 0.406: RN2.8 42.67,14.73 41.91,14.73 T4.2
N$22
  Top 0.813: T5.3 49.53,5.84 S56.1
N$23
  Top 0.813: T6.3 55.88,4.32 56.9,3.3 S56.2
N$24
  Top 0.813: S78.1 T7.3
N$25
  Top 0.813: T8.3 68.58,4.57 67.31,3.3 S78.2
N$26
  Top 0.406: RN3.2 49.02,14.73 48.26,14.73 T5.2
N$27
  Top 0.406: RN3.4 57.15,17.27 54.61,14.73 T6.2
N$28
  Top 0.406: RN3.6 62.23,16 60.96,14.73 T7.2
N$29
  Top 0.406: T8.2 RN3.8
N$30
  Top 0.406: C8.2 R4.2 86.36,43.18 | 86.36,43.18 R5.1 | RJ45.6 85.6,22.1 83.82,20.32 L2.1 80.52,20.32 80.01,20.83 80.01,26.92 81.03,27.94 83.57,27.94 86.36,30.73 86.36,43.18
N$31
  Bottom 0.406: PTC.P$1 13.72,35.05 7.87,35.05 6.6,36.32 2.03,36.32 J2.3
N$32
  Top 0.406: RN1.3 RN1.2 93.47,52.83 93.47,54.36 94.49,55.37 97.28,55.37 B1.1
N$33
  Bottom 0.406: RN1.6 97.54,34.54 B3.1
N$34  (via drill 0.3)
  Top 0.406: v76.2,32 v76.2,36.07 | v78.49,46.99 78.49,57.66 81.79,60.96 IC6.27
  Bottom 0.406: RA.1 73.66,25.15 76.2,27.69 v76.2,32 | v76.2,36.07 78.49,38.35 v78.49,46.99
N$35
  Top 0.406: RN1.5 91.44,45.21 | 91.44,45.21 97.28,45.21 B2.1 | 91.44,45.21 RN1.4
N$36
  Top 0.406: RB.1 70.61,26.67 69.85,27.43 69.85,31.5 69.6,31.75 69.6,33.27 73.15,36.83 83.06,36.83 83.82,37.59 83.82,38.61 83.06,39.37 80.77,39.37 79.25,40.89 79.25,55.88 81.79,58.42 IC6.26
N$37
  Top 0.406: 5.08,57.15 LED.K | 5.08,57.15 RLED.1 | JP2.1 5.08,57.15
N$38
  Top 0.406: RD+.2 10.16,28.7 10.67,28.19 USB.D+
N$39
  Top 0.406: RLED.2 D3.A
  Bottom 0.406: D3.A 7.62,48.51 22.35,63.25 LCD.3
N$40
  Bottom 0.813: IC1.7 31.75,40.64 35.56,36.83 D2.C 34.29,29.97 34.29,25.4 L1.1
N$41
  Top 0.406: R5.2 88.14,35.05 88.14,23.62 RJ45.7
  Bottom 0.406: R5.2 86.36,36.83 84.84,36.83 83.57,35.56 IC6.17
N$42
  Top 0.406: R4.1 82.55,33.02 IC6.16
  Bottom 0.406: RJ45.8 85.6,24.89 85.6,28.96 83.82,30.73 83.82,31.24 82.04,33.02 IC6.16
N$43  (via drill 0.3)
  Top 0.406: v76.96,26.92 76.96,21.34 82.55,15.75 88.14,15.75 RJ45.1 | v83.82,46.99 R3.2
  Bottom 0.406: 76.96,27.18 76.96,32.26 76.2,33.02 IC6.13 | v83.82,46.99 80.77,46.99 79.25,45.47 79.25,29.46 76.96,27.18 | v76.96,26.92 76.96,27.18
N$44  (via drill 0.3)
  Top 0.406: v78.49,29.72 78.74,29.46 78.74,20.57 82.04,17.27 85.6,17.27 RJ45.2
  Bottom 0.406: R2.1 83.82,49.53 80.01,49.53 77.72,47.24 77.72,38.86 74.42,35.56 IC6.12 74.68,35.56 78.49,31.75 v78.49,29.72
N$45
  Top 0.406: RD-.2 8.64,36.83 9.91,38.1 10.41,38.1 11.43,37.08 11.43,29.46 12.7,28.19 USB.D-
N$46
  Top 0.406: D4.A 18.29,20.32 JP4.1
N$47
  Top 0.406: JP3.1 85.09,4.32 86.11,3.3 RAIN.2
N$48
  Top 0.406: RLCD.1 58.67,63.25 55.63,63.25 LCD.16
N$50
  Top 0.406: C6.+ 91.44,60.71 89.41,60.71 85.34,64.77 75.69,64.77 74.42,63.5 IC6.1
N$51
  Top 0.406: IC6.14 79.5,30.48 80.77,31.75 84.58,31.75 85.09,31.24 R6.1
N$52
  Top 0.406: CX3.1 69.85,44.45 X2.1
  Bottom 0.406: IC6.24 79.25,53.34 75.44,49.53 72.14,49.53 69.09,52.58 68.07,52.58 67.31,51.82 67.31,44.96 66.8,44.45 X2.1
N$53
  Top 0.406: CX4.1 69.85,39.37 X2.2
  Bottom 0.406: CX4.1 72.39,41.91 75.44,41.91 76.2,42.67 76.2,46.74 80.26,50.8 IC6.23
N$54
  Top 0.406: R2.2 R3.1 C7.2
QH*  (via drill 0.3)
  Top 0.406: IC5.9 55.88,28.7 62.48,22.1 70.36,22.1 v74.17,18.29 | v78.23,18.29 78.23,17.02 JPEXT.8
  Bottom 0.406: v74.17,18.29 v78.23,18.29
RESET  (via drill 0.3)
  Top 0.406: B0.3 12.19,12.7 18.29,12.7 B0.4 18.54,12.95 21.34,12.95 24.13,15.75 24.38,15.75 25.4,16.76 25.4,17.78 24.13,19.05 23.11,19.05 18.03,24.13 18.03,34.04 IC7.1 | RRST.2 IC4.1 | JP1.10 73.91,27.94 74.93,26.92 74.93,20.83 76.2,19.56 v76.2,14.73
  Bottom 0.406: JP1.10 72.39,29.21 72.39,38.86 74.17,40.64 IC6.10 | IC7.1 16.51,36.32 22.86,42.67 22.86,43.69 29.97,50.8 RRST.2 | v76.2,14.73 76.2,12.19 73.15,9.14 21.08,9.14 18.54,11.68 18.54,12.7 B0.4
RXD  (via drill 0.3)
  Top 0.406: v42.16,43.94 43.94,43.94 v45.47,42.42 | v49.53,41.66 v52.32,38.86 | v54.61,34.54 56.13,33.02 60.71,33.02 v61.47,32.26
  Bottom 0.406: IC4.2 38.1,48.51 39.37,47.24 39.37,46.74 v42.16,43.94 | v45.47,42.42 46.23,42.42 46.99,43.18 48.01,43.18 v49.53,41.66 | v52.32,38.86 54.61,36.58 v54.61,34.54 | v61.47,32.26 65.79,27.94 JP1.6
SCK  (via drill 0.3)
  Top 0.406: IC8.SCK 12.45,49.28 13.46,49.28 19.05,43.69 IC7.7 19.05,42.42 25.4,36.07 25.4,35.05 v23.88,33.53 | IC4.19 61.98,54.86 61.98,54.61 64.77,51.82 64.77,49.78 67.56,46.99 72.9,46.99 74.17,45.72 IC6.8 | v69.85,16 71.88,13.97 88.9,13.97 89.66,14.73 89.66,50.29 87.88,52.07 v80.77,52.07
  Bottom 0.406: v23.88,33.53 23.88,32.51 36.83,19.56 36.83,16.76 37.59,16 v69.85,16 | v80.77,52.07 80.26,51.56 80.01,51.56 74.17,45.72 IC6.8
SCL  (via drill 0.3)
  Top 0.406: IC4.28 35.56,57.66 37.85,55.37 v51.56,55.37 | JP1.3 63.5,26.16 64.77,27.43 64.77,32 v62.99,33.78
  Bottom 0.406: v51.56,55.37 51.56,54.86 54.61,51.82 54.61,49.53 54.36,49.28 54.36,48.77 54.86,48.26 56.13,48.26 57.15,47.24 57.15,44.45 57.28,44.32 | 57.28,44.32 IC3.6 | v62.99,33.78 57.91,33.78 57.15,34.54 57.15,44.2 57.28,44.32
SDA  (via drill 0.3)
  Top 0.406: v50.29,42.16 52.07,42.16 52.83,41.4 59.18,41.4 IC3.5 | JP1.1 60.96,26.16 62.23,27.43 v62.23,34.54
  Bottom 0.406: IC4.27 44.45,52.07 44.45,48.51 45.72,47.24 45.72,46.74 v50.29,42.16 | v62.23,34.54 62.23,41.91 IC3.5
TXD  (via drill 0.3)
  Top 0.406: v44.7,38.35 46.99,36.07 48.01,36.07 v49.02,37.08
  Bottom 0.406: IC4.3 40.64,48.51 44.7,44.45 v44.7,38.35 | v49.02,37.08 49.53,37.08 54.36,32.26 59.18,32.26 JP1.4
VCC
  Top 0.406: 83.82,55.88 88.9,55.88 RN1.1 | 83.82,55.88 IC6.25 81.79,55.88 80.01,54.1 80.01,44.96 81.79,43.18 IC6.20 82.04,43.18 82.04,40.64 IC6.19 | 83.82,55.88 83.82,61.72 82.04,63.5 IC6.28 | IC4.7 50.8,51.56 55.88,56.64 IC4.20 | C3.+ 42.93,42.16 47.5,37.59 IC2.3 | R7.2 10.41,46.74 10.41,47.75 6.35,51.82 6.35,56.9 7.11,57.66 8.13,57.66 8.38,57.4 12.19,57.4 IC8.VDD | IC5.16 37.59,30.48 27.43,20.32 D4.C 22.86,21.59 22.86,36.07 16.51,42.42 IC7.8
  Bottom 0.406: 70.61,20.32 70.61,14.48 JPEXT.1 | IC6.19 81.79,40.64 80.01,38.86 80.01,32.26 81.79,30.48 IC6.15 81.53,30.48 71.37,20.32 70.61,20.32 | 70.61,20.32 L2.2 66.8,20.32 62.23,24.89 62.23,26.67 JP1.2 55.88,27.94 IC5.10 53.34,31.75 47.75,37.34 IC2.3 47.5,37.34 | C3.+ 42.93,44.7 C4.1 39.37,48.26 39.37,51.82 38.61,52.58 38.1,52.58 32.26,58.42 RRST.1 | 47.5,37.34 IC3.8 53.09,43.18 50.29,45.97 50.29,47.5 50.8,48.01 IC4.7 | IC7.8 13.97,43.18 R7.2 | 47.5,37.34 46.23,37.34 43.43,34.54 40.13,34.54 38.1,32.51 IC5.16
VIN
  Top 0.406: LCD.15 52.83,63.5 51.31,65.02 21.59,65.02 20.07,63.5 LCD.2 | 29.21,32.51 29.21,25.4 L1.2 | 29.21,32.51 IC1.1 | C2.+ 42.93,34.04 41.15,32.26 36.32,32.26 36.07,32.51 29.21,32.51
  Bottom 0.406: LED.A 16.26,59.69 19.81,63.25 LCD.2 | C2.+ 44.96,37.08 IC2.2 48.77,39.62 51.05,41.91 51.05,42.42 49.53,43.94 49.53,51.82 49.78,52.07 49.78,54.1 49.53,54.36 49.53,59.44 52.83,62.74 52.83,63.25 LCD.15 | JPEXT.7 79.25,12.7 74.93,8.38 20.83,8.38 17.02,12.19 17.02,17.78 20.45,21.21 | 20.45,21.21 24.64,25.4 L1.2 | USB.VBUS 12.95,25.65 16,25.65 20.45,21.21

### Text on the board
tNames: OpenSprinkler (v1.2u) | 46045_A | Rayshobby, Mar 2012 | PWR | SEN | 1N4148 | MEGA328 | RFM12B | ENC28J60 | TINY45 | LM2574 | 24LC | 1N5819 | VCC TXD RXD GND RST | 100u | USB | 74HC595 | 1N4001 | SDA SCL D2 D3 A1 | RJ45 | Din CLK LAT Dout | BAT | GND | AC IN | VCC GND GND VIN | GND | RAIN | SEN | 1 | 2 | 3 | 4 | 5 | 6 | 7 | 8
BoxDim: Serpac WM-032RC Enclosure | All units are in inch | Left | Right | Front | 0.14 | 0.32 | 1.28 | 0.91 | 0.32 | 1.0 | 0.26 | 0.4 | 0.29 | 3.25 | 0.45 | 0.7 | 0.53 | 0.4 | 0.32 | 0.63 | Bottom | 1.28 | 0.32 | 1.6 | 1.6 | 4.38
